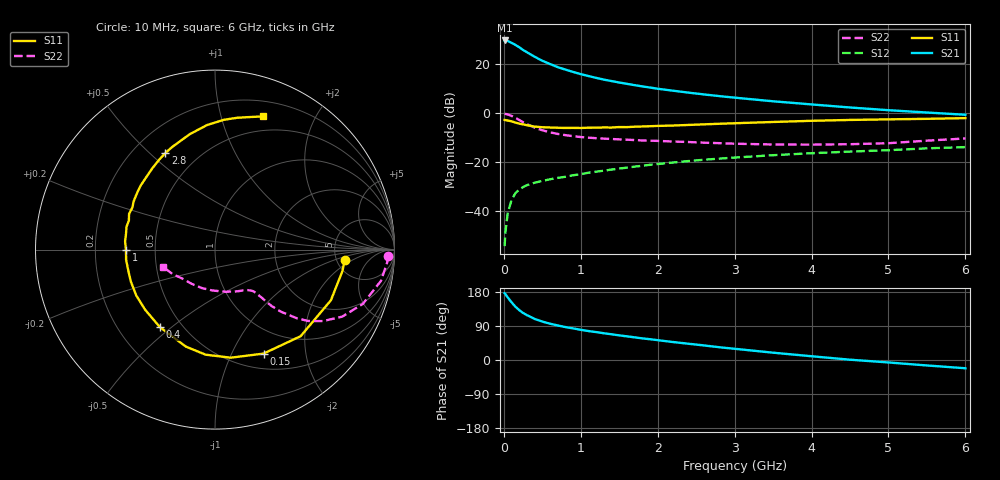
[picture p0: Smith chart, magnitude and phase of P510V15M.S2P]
! SIEMENS Small Signal Semiconductors
! BFP183
! Si NPN RF Bipolar Junction Transistor in SOT143
! VCE = 10 V  IC = 15 mA
! Common Emitter S-Parameters:  March  1996
# GHz  S  MA  R  50
!  f  S11  S21  S12  S22
! GHz  MAG  ANG  MAG  ANG  MAG  ANG  MAG  ANG
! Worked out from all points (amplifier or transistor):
!   36 points, 10 MHz to 6 GHz, reference 50 ohm
!   highest |S21| = 29.7 dB at 10 MHz (marker M1)
!   |S21| within 3 dB of that: start of sweep to 209.8 MHz
!   unconditionally stable (mu >= 1): 1.129 GHz to 5.904 GHz
!   at 250 MHz: K = 0.37, MSG = 28.0 dB, |S12| = -30.3 dB
!   at 1.4 GHz: K = 1.08, MAG = 16.4 dB, |S12| = -23.1 dB
!   at 6 GHz: K = 0.99, MSG = 6.6 dB, |S12| = -13.9 dB
!   S11 on the Smith chart (normalised r, x): 10 MHz: 5.94, -1.39; 150 MHz: 0.68, -1.33; 400 MHz: 0.38, -0.46; 1 GHz: 0.34, -0.00; 2.8 GHz: 0.33, +0.56; 6 GHz: 0.35, +1.36
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0.01  0.7251 -4.4  30.58 176.3  0.0019 76.1  0.9648 -2.0
0.02  0.7202 -9.5  30.38 173.9  0.0036 81.1  0.962 -4.3
0.05  0.7048 -23.6  29.81 165.2  0.0089 76.5  0.9408 -10.7
0.1  0.6786 -45.3  27.38 152.3  0.0167 67.0  0.8772 -20.2
0.15  0.6394 -65.0  24.83 140.8  0.0231 60.4  0.801 -27.8
0.2  0.6086 -81.7  22.19 131.6  0.0273 55.3  0.7218 -33.5
0.25  0.5878 -95.1  19.53 124.2  0.0307 51.7  0.6531 -37.5
0.3  0.5644 -106.7  17.55 118.4  0.0336 49.8  0.5949 -40.0
0.4  0.5299 -125.4  14.21 108.4  0.0377 46.5  0.5046 -43.3
0.5  0.5137 -139.3  11.75 101.4  0.0411 44.9  0.4453 -44.9
0.6  0.5077 -149.9  10.09 95.8  0.0443 44.9  0.4044 -45.5
0.7  0.5015 -159.3  8.715 91.1  0.0473 45.3  0.3753 -45.8
0.8  0.497 -166.9  7.753 86.9  0.0499 45.3  0.3541 -46.2
1  0.4962 -179.7  6.26 79.7  0.0562 46.3  0.324 -47.0
1.1  0.503 174.7  5.729 76.4  0.0604 46.7  0.3142 -47.5
1.5  0.5184 157.5  4.223 65.0  0.0736 46.7  0.29 -51.1
2.2  0.5566 133.4  2.868 47.4  0.0976 43.9  0.2624 -62.3
2.8  0.6048 117.3  2.226 33.7  0.1172 39.5  0.2431 -75.4
3.5  0.6584 102.3  1.744 19.3  0.1377 34.3  0.2282 -93.9
4.5  0.7244 86.2  1.302 0.8  0.1633 25.9  0.2312 -124.8
5.5  0.7635 75.3  1.028 -14.4  0.1902 19.0  0.273 -150.1
6  0.7886 70.2  0.924 -21.8  0.2017 14.7  0.3032 -161.2
